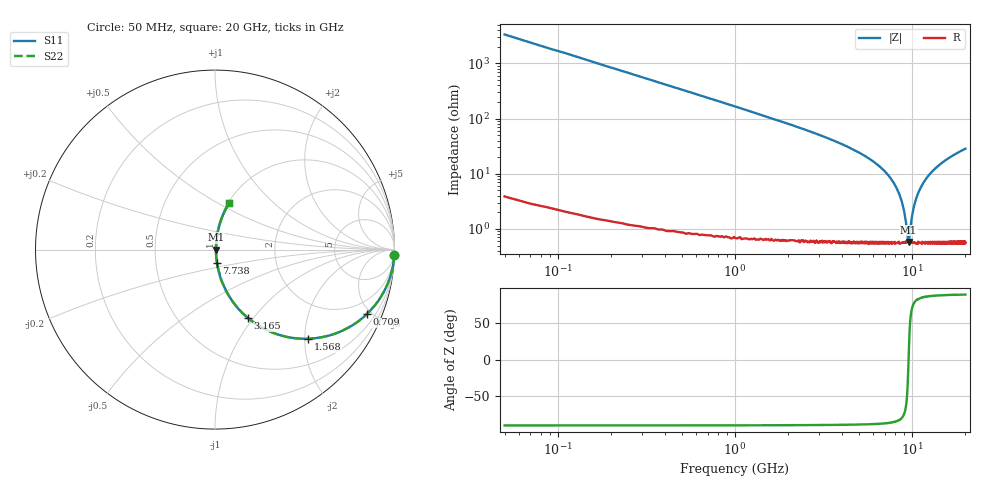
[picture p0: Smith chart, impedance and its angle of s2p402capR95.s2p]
! AVX Thin Film Operation		Date: September 2011
! Description: Accu-P® Series, Thin Film, SMD, RF Capacitor
! Part Number: 04021JR95ZBW/STR
! 50 MHz  -  20 GHz
! Serial Measurements
# MHZ S MA R 50
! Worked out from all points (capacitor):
!   1000 points, 50 MHz to 20 GHz, reference 50 ohm
!   read as one part in series: C = 950 fF near 149.8 MHz
!   lowest |Z| = 582 mohm at 9.556 GHz (marker M1)
!   series resonance near 9.549 GHz, so ESL is about 290 pH
!   S11 on the Smith chart (normalised r, x): 50 MHz: 0, -67; 709 MHz: 1.02, -4.70; 1.568 GHz: 1.01, -2.08; 3.165 GHz: 1.01, -0.94; 7.738 GHz: 1.01, -0.15; 20 GHz: 1.01, +0.57
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50  1 -1.7  0.03 88.2  0.03 88.2  1 -1.7
189.79  0.993 -6.5  0.113 83.4  0.113 83.4  0.993 -6.5
309.61  0.983 -10.5  0.182 79.4  0.182 79.4  0.983 -10.5
489.339  0.959 -16.3  0.281 73.5  0.281 73.5  0.959 -16.3
709.009  0.919 -23.0  0.391 66.8  0.391 66.8  0.919 -23.0
1567.718  0.719 -43.7  0.691 45.9  0.691 45.9  0.719 -43.7
2306.607  0.562 -55.3  0.822 34.2  0.822 34.2  0.562 -55.3
3165.315  0.424 -64.2  0.9 25.1  0.9 25.1  0.424 -64.2
3384.985  0.395 -66.0  0.913 23.3  0.913 23.3  0.395 -66.0
6700  0.125 -80.3  0.987 7.2  0.987 7.2  0.125 -80.3
7738.438  0.074 -81.5  0.992 4.2  0.992 4.2  0.074 -81.5
8377.477  0.046 -80.4  0.993 2.6  0.993 2.6  0.046 -80.4
8836.787  0.028 -76.8  0.994 1.6  0.994 1.6  0.028 -76.8
9116.366  0.017 -70.1  0.994 0.9  0.994 0.9  0.017 -70.1
9455.856  0.006542 -31.5  0.994 0.2  0.994 0.2  0.006542 -31.5
9555.706  0.005573 2.4  0.994 -0.0  0.994 -0.0  0.005573 2.4
10034.99  0.018 71.2  0.994 -1.0  0.994 -1.0  0.018 71.2
10554.2  0.035 78.9  0.994 -2.0  0.994 -2.0  0.035 78.9
11233.18  0.057 81.2  0.993 -3.3  0.993 -3.3  0.057 81.2
13350  0.118 80.5  0.987 -6.8  0.987 -6.8  0.118 80.5
16684.99  0.201 76.8  0.974 -11.6  0.974 -11.6  0.201 76.8
20000  0.272 73.1  0.957 -15.8  0.957 -15.8  0.272 73.1
